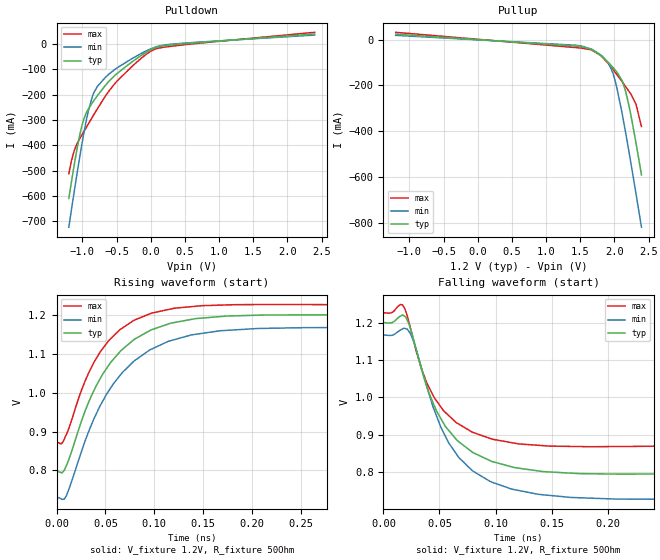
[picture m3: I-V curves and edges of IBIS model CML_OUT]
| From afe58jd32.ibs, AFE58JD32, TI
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|   Model
[Model]   CML_OUT
Model_type   Output
Polarity   Non-Inverting
Vmeas = 1
Vref = 1.2
Cref = 1pF
Rref = 50
|   typ   min   max
C_comp   1.531pF   1.472pF   1.554pF
[Voltage Range]   1.2   1.14   1.26
[Temperature Range]   25   85   -40
[Pullup Reference]   1.2   1.14   1.26
[Pulldown Reference]   -0   -0   -0
[Power Clamp Reference]   1.2   1.14   1.26
[GND Clamp Reference]   -0   -0   -0
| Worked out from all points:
|   slope of the pulldown table from 0 to 0.18 V, typ, clamps not added: 12 ohm
|   slope of the pullup table from 0 to 0.18 V, typ, clamps not added: 50.5 ohm
|   falling waveform, V_fixture 1.2V, R_fixture 50Ohm: 20-80 % time 38.4ps typ, 40.9ps min, 34.5ps max; typ from 1.2 V to 0.798 V
|   rising waveform, V_fixture 1.2V, R_fixture 50Ohm: 20-80 % time 51.9ps typ, 57.1ps min, 44.9ps max; typ from 0.798 V to 1.2 V
[Pulldown]
|   Voltage   I(typ)   I(min)   I(max)
-1.2V     -610mA     -723.2mA   -512.2mA
-1.157V   -536.1mA   -645.9mA   -455.8mA
-1.121V   -477mA     -582.6mA   -420.8mA
-1.052V   -375.3mA   -466.2mA   -379.6mA
-1.009V   -323.4mA   -396.6mA   -359.2mA
-915.6mV  -257.1mA   -265.5mA   -316.1mA
-854.4mV  -231.4mA   -206.1mA   -288.2mA
-782.4mV  -204.1mA   -167.5mA   -255.8mA
-519.6mV  -122.3mA   -98.9mA    -154mA
-105.6mV  -38.84mA   -32.2mA    -48.47mA
99.6mV    -11.72mA   -9.092mA   -17.01mA
2.396V    39.76mA    35.59mA    46.37mA
[Pullup]
|   Voltage   I(typ)   I(min)   I(max)
-1.2V     23.77mA    18.68mA    31.88mA
1.457V    -28.96mA   -25.37mA   -35.34mA
1.658V    -41.56mA   -40.76mA   -44.41mA
1.799V    -67.81mA   -66.56mA   -69.32mA
1.91V     -99.25mA   -100.8mA   -104.4mA
1.975V    -120.3mA   -143mA     -128.6mA
2.044V    -144.7mA   -220.2mA   -155.6mA
2.13V     -192.3mA   -349.1mA   -190.9mA
2.166V    -227.3mA   -408.3mA   -205.8mA
2.22V     -297.2mA   -500.7mA   -228.5mA
2.317V    -452.1mA   -673.9mA   -283.3mA
2.396V    -590.8mA   -819.1mA   -379.8mA
[Ramp]
R_load = 50
|   typ   min   max
dV/dt_r   0.241315/5.19251e-11   0.262488/5.71308e-11   0.212329/4.49008e-11
dV/dt_f   0.241329/3.84268e-11   0.262506/4.08768e-11   0.212339/3.44975e-11
[Falling Waveform]
V_fixture = 1.2V
V_fixture_min = 1.14V
V_fixture_max = 1.26V
R_fixture = 50Ohm
C_fixture = 0F
|   Time   V(typ)   V(min)   V(max)
0s        1.2V       1.167V     1.227V
15.05ps   1.217V     1.18V      1.248V
21.37ps   1.205V     1.182V     1.217V
33.58ps   1.08V      1.082V     1.079V
45.05ps   979.7mV    968.2mV    1V
58.18ps   911.6mV    878.2mV    951.4mV
67.25ps   881mV      838.9mV    928.2mV
95.51ps   830mV      774.4mV    889.7mV
167.4ps   797.1mV    732.2mV    868.6mV
400ps     798mV      729.7mV    872.6mV
[Rising Waveform]
V_fixture = 1.2V
V_fixture_min = 1.14V
V_fixture_max = 1.26V
R_fixture = 50Ohm
C_fixture = 0F
|   Time   V(typ)   V(min)   V(max)
0s        798mV      729.7mV    872.6mV
5.065ps   794.4mV    726.4mV    869mV
10ps      812.1mV    734.4mV    892.5mV
33.58ps   979.8mV    904.7mV    1.055V
53.51ps   1.071V     1.005V     1.135V
79.49ps   1.137V     1.082V     1.187V
114.5ps   1.177V     1.133V     1.214V
167.4ps   1.196V     1.16V      1.226V
206.2ps   1.2V       1.166V     1.227V
400ps     1.2V       1.167V     1.227V
